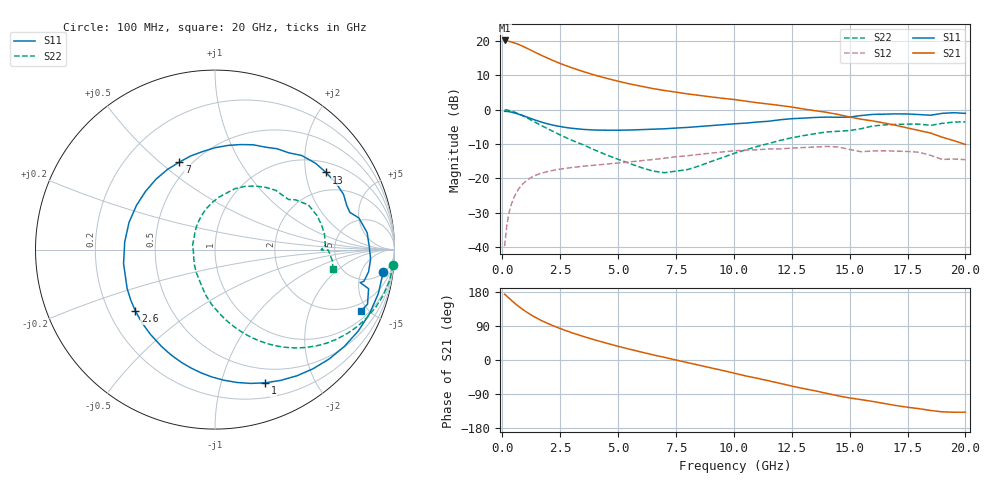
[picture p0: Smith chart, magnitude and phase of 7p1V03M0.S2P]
! Infineon Technologies  Discrete & RF Semiconductors
! bfp620
! VCE =  1.0 V,  IC =  3.0 mA
! Common Emitter S-Parameters:  Sep 2002
# GHz  S  MA  R  50
!  f  S11  S21  S12  S22
! GHz  MAG  ANG  MAG  ANG  MAG  ANG  MAG  ANG
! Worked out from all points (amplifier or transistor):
!   59 points, 100 MHz to 20 GHz, reference 50 ohm
!   highest |S21| = 20.1 dB at 100 MHz (marker M1)
!   |S21| within 3 dB of that: start of sweep to 1.282 GHz
!   unconditionally stable (mu >= 1): 5.428 GHz to 12.29 GHz; 14.46 GHz to 15.67 GHz; 17.09 GHz to end of sweep
!   at 1 GHz: K = 0.22, MSG = 19.5 dB, |S12| = -20.9 dB
!   at 5.5 GHz: K = 1.01, MAG = 10.8 dB, |S12| = -15.2 dB
!   at 20 GHz: K = 1.56, MAG = -2.2 dB, |S12| = -14.6 dB
!   S11 on the Smith chart (normalised r, x): 100 MHz: 5, -13; 1 GHz: 0.35, -1.39; 2.6 GHz: 0.31, -0.31; 7 GHz: 0.43, +0.58; 13 GHz: 1.31, +2.60; 20 GHz: 1.47, -4.53
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0.1  0.9455 -7.6  10.16 173.7  0.0103 86.3  0.9963 -5.0
0.3  0.9324 -22.4  9.853 162.7  0.0324 77.9  0.9729 -14.8
0.5  0.9004 -36.8  9.418 151.8  0.0523 69.5  0.9284 -24.0
0.6  0.8809 -43.8  9.167 146.7  0.0613 65.6  0.9015 -28.4
0.8  0.8382 -57.0  8.612 137.2  0.0771 58.3  0.8423 -36.3
1  0.7935 -69.3  8.018 128.5  0.0901 51.8  0.7801 -43.4
1.3  0.7294 -86.1  7.145 117.0  0.1052 43.7  0.6892 -52.5
1.7  0.6578 -105.9  6.156 103.9  0.119 35.4  0.5841 -62.3
2.2  0.5939 -127.2  5.178 90.3  0.1308 27.7  0.4805 -72.2
2.6  0.5604 -142.3  4.562 80.8  0.1377 22.9  0.4133 -79.3
3  0.5356 -156.0  4.068 72.0  0.1436 18.8  0.3594 -85.7
3.5  0.5155 -171.2  3.579 62.1  0.1501 14.6  0.3073 -93.4
4  0.5049 175.2  3.176 53.0  0.1555 10.8  0.2582 -101.6
5  0.5021 150.6  2.593 36.1  0.1675 4.9  0.1891 -117.9
7  0.5264 112.1  1.902 7.0  0.1962 -6.5  0.1209 -173.5
8.5  0.5678 89.9  1.615 -13.7  0.2233 -17.0  0.1514 137.0
10.5  0.6361 63.8  1.332 -41.8  0.2568 -35.0  0.2585 94.5
13  0.7531 34.8  1.024 -75.3  0.2809 -57.5  0.4183 57.8
13.5  0.7692 29.0  0.965 -81.3  0.2848 -62.5  0.446 51.2
15  0.7797 15.4  0.783 -100.2  0.2635 -82.4  0.4964 34.2
17  0.8686 -3.5  0.591 -120.1  0.2489 -93.0  0.61 12.7
20  0.8828 -22.7  0.311 -137.7  0.1871 -110.5  0.6652 -9.4
